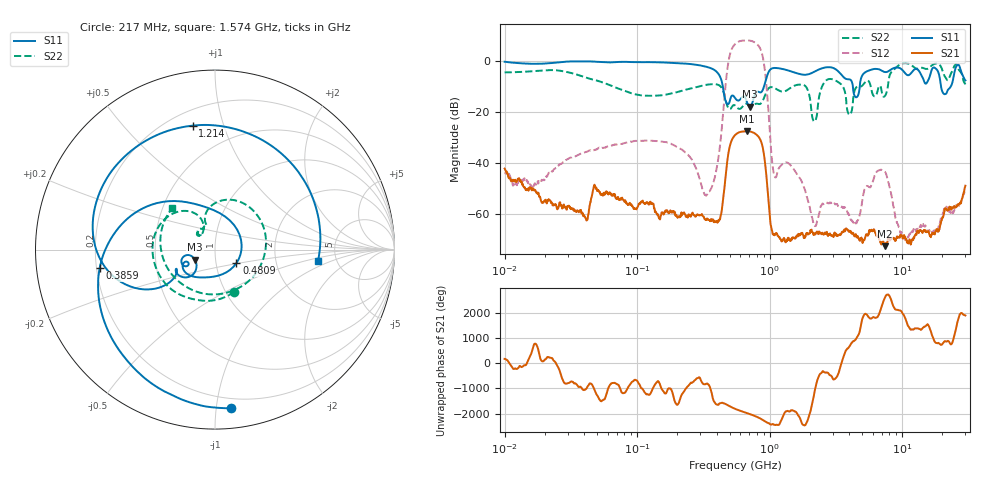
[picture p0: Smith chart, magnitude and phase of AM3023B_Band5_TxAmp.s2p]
# Hz S DB R 50.0
!freq dBS11 angS11 dBS21 angS21 dBS12 angS12 dBS22 angS22
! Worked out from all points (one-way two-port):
!   1601 points, 10 MHz to 30 GHz, reference 50 ohm
!   highest |S21| = -27.68 dB at 672.5 MHz (marker M1); lowest = -72.7 dB at 7.39 GHz (marker M2)
!   lowest |S11| = -18.1 dB at 707 MHz (marker M3), VSWR 1.29, Z = 39.7 - j4.6 ohm
!   |S11| at or under -10 dB: 443 MHz to 907.6 MHz (464.7 MHz wide, 68.8 % of centre); 4.244 GHz to 4.784 GHz (539.8 MHz wide, 12 % of centre); 19.63 GHz to 23.32 GHz (3.695 GHz wide, 17.2 % of centre)
!   |S22| runs from -23.8 to -0.9 dB; largest |S21 - S12| = 2.5
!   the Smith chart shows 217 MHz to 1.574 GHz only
!   S11 on the Smith chart (normalised r, x): 217 MHz: 0.13, -1.10; 385.9 MHz: 0.21, -0.08; 480.9 MHz: 1.25, -0.19; 1.214 GHz: 0.29, +0.79; 1.574 GHz: 3.58, -0.71
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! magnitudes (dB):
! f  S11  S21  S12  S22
! 10 MHz  -0.4  -42.3  -43.7  -4.5
! 38.04 MHz  -0.2  -59.6  -36.4  -6.0
! 48.61 MHz  -0.4  -49.5  -34.9  -7.6
! 144.7 MHz  -0.6  -61.0  -31.6  -13.6
! 217 MHz  -1.0  -60.7  -34.8  -11.8
! 325.5 MHz  -2.2  -62.2  -52.5  -9.5
! 385.9 MHz  -3.7  -63.3  -45.6  -9.2
! 480.9 MHz  -17.0  -38.6  -2.8  -17.9
! 547.7 MHz  -14.6  -29.2  6.5  -17.5
! 672.5 MHz  -16.1  -27.7  8.0  -16.9
! 707 MHz  -18.1  -27.7  7.9  -17.5
! 876.7 MHz  -12.0  -32.9  2.7  -16.2
! 1.066 GHz  -2.9  -67.9  -43.2  -10.5
! 1.214 GHz  -3.1  -70.1  -41.2  -12.0
! 1.574 GHz  -4.8  -69.5  -43.7  -9.6
! 2.084 GHz  -4.8  -67.2  -61.3  -21.2
! 2.73 GHz  -2.5  -68.4  -55.8  -7.4
! 4.458 GHz  -14.3  -68.3  -63.8  -10.7
! 7.39 GHz  -4.4  -72.7  -43.6  -13.9
! 7.926 GHz  -4.0  -69.4  -48.2  -7.3
! 10.7 GHz  -5.3  -70.1  -69.3  -0.9
! 30 GHz  -7.7  -49.0  -50.7  -9.3
